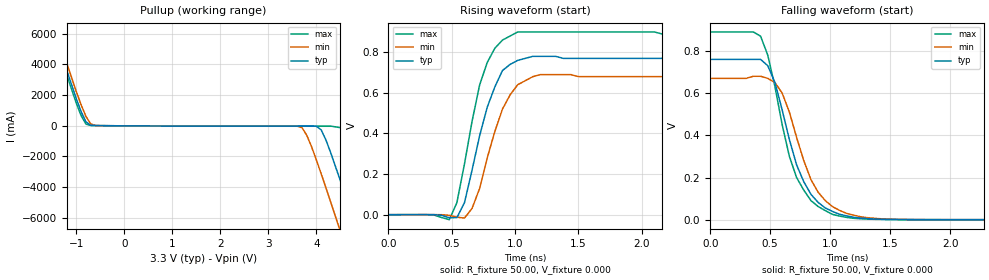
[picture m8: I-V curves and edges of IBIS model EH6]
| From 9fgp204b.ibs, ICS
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|   Model EH6
[Model]   EH6
Model_type   Open_source
Polarity   Inverting
Vmeas =   1.50V
Rref =  50.000
Vref =   1.50V
C_comp   3.40pF   2.85pF   3.95pF
[Temperature Range]   27.00   70.00   0.000
[Voltage Range]   3.30V   3.00V   3.70V
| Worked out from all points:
|   slope of the pullup table from 0 to 0.495 V, typ, clamps not added: 53.8 ohm
|   rising waveform, R_fixture 50.00, V_fixture 0.000: 20-80 % time 196ps typ, 198ps min, 182ps max; typ from 0 V to 0.77 V
|   falling waveform, R_fixture 50.00, V_fixture 0.000: 20-80 % time 249ps typ, 253ps min, 235ps max; typ from 0.76 V to 0 V
[Pullup]
| voltage   I(typ)   I(min)   I(max)
-3.3V     24.07A     24.5A      23.8A
-1.5V     6.41A      6.88A      6.12A
-1V       1.75A      2.22A      1.46A
-800mV    260mA      610mA      110mA
-600mV    15.6mA     18.69mA    16.79mA
3.7V      -15.37mA   -120mA     -17.88mA
4.1V      -260mA     -3.12A     -17.91mA
4.5V      -3.57A     -6.88A     -120mA
4.7V      -5.46A     -8.81A     -1.47A
4.9V      -7.39A     -10.75A    -3.28A
5.3V      -11.28A    -14.66A    -7.1A
6.6V      -24.09A    -27.49A    -19.87A
[Ramp]
| variable   typ   min   max
dV/dt_r   0.46/0.19n   0.41/0.20n   0.54/0.18n
dV/dt_f   0.46/0.24n   0.40/0.25n   0.53/0.23n
R_load = 50.00
[Rising Waveform]
R_fixture = 50.00
V_fixture = 0.000
V_fixture_min = 0.000
V_fixture_max = 0.000
| time   V(typ)   V(min)   V(max)
0s        -29uV      -27.13uV   -30.44uV
480ps     -15.1mV    -3.18mV    -24.66mV
540ps     -14.67mV   -12.36mV   58.89mV
600ps     58.91mV    -16.72mV   250mV
720ps     390mV      130mV      640mV
780ps     530mV      280mV      750mV
900ps     710mV      520mV      860mV
1.02ns    760mV      640mV      900mV
1.2ns     780mV      690mV      900mV
3ns       770mV      680mV      890mV
[Falling Waveform]
R_fixture = 50.00
V_fixture = 0.000
V_fixture_min = 0.000
V_fixture_max = 0.000
| time   V(typ)   V(min)   V(max)
0s        760mV      670mV      890mV
420ps     760mV      680mV      870mV
480ps     730mV      670mV      780mV
540ps     650mV      650mV      630mV
600ps     520mV      600mV      450mV
720ps     260mV      390mV      200mV
840ps     120mV      190mV      90.37mV
1.02ns    38.99mV    61.61mV    24.92mV
1.44ns    1.98mV     3.67mV     1.04mV
3ns       6.74uV     -14.21uV   2.93uV
